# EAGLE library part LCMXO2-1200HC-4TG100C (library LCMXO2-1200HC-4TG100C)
FPGA - Field Programmable Gate Array 1280 LUTs 80 I/O 3.3V -4 SPD Source: Datasheet
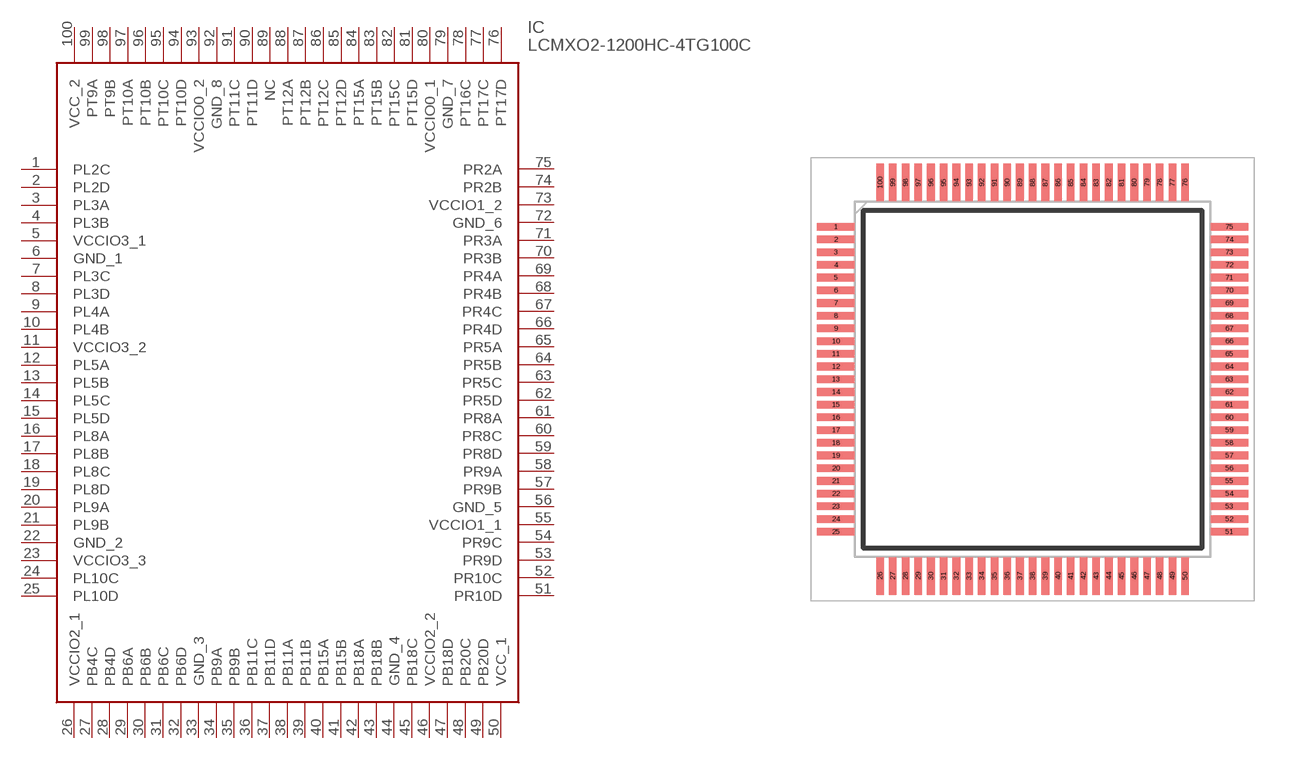
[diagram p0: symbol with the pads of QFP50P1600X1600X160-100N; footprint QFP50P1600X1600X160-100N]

Designator prefix IC

## LCMXO2-1200HC-4TG100C (Arrow_Part_Number: LCMXO2-1200HC-4TG100C; Arrow_Price-Stock: https://www.arrow.com/en/products/lcmxo2-1200hc-4tg100c/lattice-semiconductor?region=europe; Description: FPGA - Field Programmable Gate Array 1280 LUTs 80 I/O 3.3V -4 SPD; Height: 1.6mm; Manufacturer_Name: Lattice Semiconductor; Manufacturer_Part_Number: LCMXO2-1200HC-4TG100C)  [QFP50P1600X1600X160-100N]
1  PL2C
2  PL2D
3  PL3A
4  PL3B
5  VCCIO3_1  pwr
6  GND_1  pwr
7  PL3C
8  PL3D
9  PL4A
10  PL4B
11  VCCIO3_2  pwr
12  PL5A
13  PL5B
14  PL5C
15  PL5D
16  PL8A
17  PL8B
18  PL8C
19  PL8D
20  PL9A
21  PL9B
22  GND_2  pwr
23  VCCIO3_3  pwr
24  PL10C
25  PL10D
26  VCCIO2_1  pwr
27  PB4C
28  PB4D
29  PB6A
30  PB6B
31  PB6C
32  PB6D
33  GND_3  pwr
34  PB9A
35  PB9B
36  PB11C
37  PB11D
38  PB11A
39  PB11B
40  PB15A
41  PB15B
42  PB18A
43  PB18B
44  GND_4  pwr
45  PB18C
46  VCCIO2_2  pwr
47  PB18D
48  PB20C
49  PB20D
50  VCC_1  pwr
51  PR10D
52  PR10C
53  PR9D
54  PR9C
55  VCCIO1_1  pwr
56  GND_5  pwr
57  PR9B
58  PR9A
59  PR8D
60  PR8C
61  PR8A
62  PR5D
63  PR5C
64  PR5B
65  PR5A
66  PR4D
67  PR4C
68  PR4B
69  PR4A
70  PR3B
71  PR3A
72  GND_6  pwr
73  VCCIO1_2  pwr
74  PR2B
75  PR2A
76  PT17D
77  PT17C
78  PT16C
79  GND_7  pwr
80  VCCIO0_1  pwr
81  PT15D
82  PT15C
83  PT15B
84  PT15A
85  PT12D
86  PT12C
87  PT12B
88  PT12A
89  NC  nc
90  PT11D
91  PT11C
92  GND_8  pwr
93  VCCIO0_2  pwr
94  PT10D
95  PT10C
96  PT10B
97  PT10A
98  PT9B
99  PT9A
100  VCC_2  pwr

## Footprint QFP50P1600X1600X160-100N (pad centres in mm)
100-Pin TQFP Package Option 1: MachXO2, MachXOTM, ispMACH&reg; 4000
smd 1.475 x 0.3: 1 -7.738,6; 2 -7.738,5.5; 3 -7.738,5; 4 -7.738,4.5; 5 -7.738,4; 6 -7.738,3.5; 7 -7.738,3; 8 -7.738,2.5; 9 -7.738,2; 10 -7.738,1.5; 11 -7.738,1; 12 -7.738,0.5; 13 -7.738,0; 14 -7.738,-0.5; 15 -7.738,-1; 16 -7.738,-1.5; 17 -7.738,-2; 18 -7.738,-2.5; 19 -7.738,-3; 20 -7.738,-3.5; 21 -7.738,-4; 22 -7.738,-4.5; 23 -7.738,-5; 24 -7.738,-5.5; 25 -7.738,-6; 51 7.738,-6; 52 7.738,-5.5; 53 7.738,-5; 54 7.738,-4.5; 55 7.738,-4; 56 7.738,-3.5; 57 7.738,-3; 58 7.738,-2.5; 59 7.738,-2; 60 7.738,-1.5; 61 7.738,-1; 62 7.738,-0.5; 63 7.738,0; 64 7.738,0.5; 65 7.738,1; 66 7.738,1.5; 67 7.738,2; 68 7.738,2.5; 69 7.738,3; 70 7.738,3.5; 71 7.738,4; 72 7.738,4.5; 73 7.738,5; 74 7.738,5.5; 75 7.738,6
smd 0.3 x 1.475: 26 -6,-7.738; 27 -5.5,-7.738; 28 -5,-7.738; 29 -4.5,-7.738; 30 -4,-7.738; 31 -3.5,-7.738; 32 -3,-7.738; 33 -2.5,-7.738; 34 -2,-7.738; 35 -1.5,-7.738; 36 -1,-7.738; 37 -0.5,-7.738; 38 0,-7.738; 39 0.5,-7.738; 40 1,-7.738; 41 1.5,-7.738; 42 2,-7.738; 43 2.5,-7.738; 44 3,-7.738; 45 3.5,-7.738; 46 4,-7.738; 47 4.5,-7.738; 48 5,-7.738; 49 5.5,-7.738; 50 6,-7.738; 76 6,7.738; 77 5.5,7.738; 78 5,7.738; 79 4.5,7.738; 80 4,7.738; 81 3.5,7.738; 82 3,7.738; 83 2.5,7.738; 84 2,7.738; 85 1.5,7.738; 86 1,7.738; 87 0.5,7.738; 88 0,7.738; 89 -0.5,7.738; 90 -1,7.738; 91 -1.5,7.738; 92 -2,7.738; 93 -2.5,7.738; 94 -3,7.738; 95 -3.5,7.738; 96 -4,7.738; 97 -4.5,7.738; 98 -5,7.738; 99 -5.5,7.738; 100 -6,7.738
